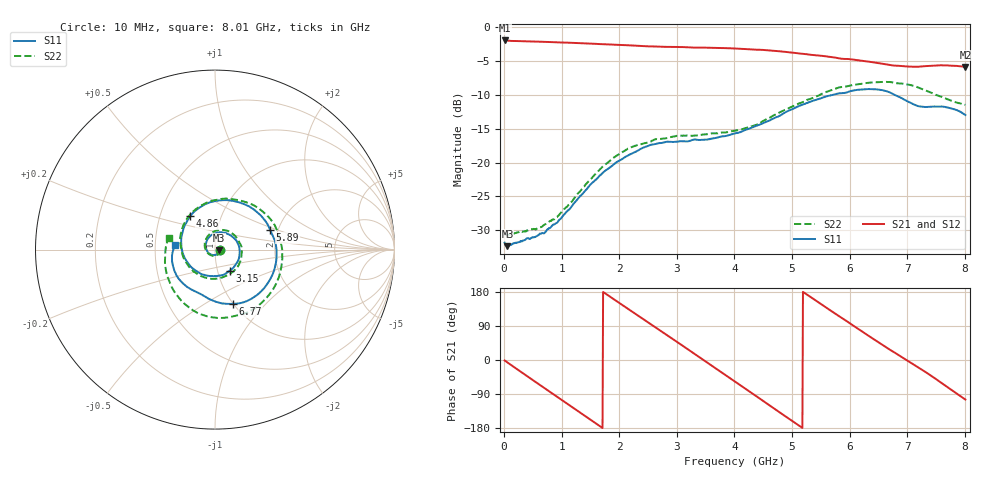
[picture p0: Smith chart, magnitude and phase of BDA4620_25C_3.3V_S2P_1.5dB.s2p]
!Agilent Technologies,E5071B,MY42404982,A.09.10
!Date: Wed May 06 08:56:16 2026
!Data & Calibration Information:
!Freq	S11:SOLT2(ON)	S21:SOLT2(ON)	S12:SOLT2(ON)	S22:SOLT2(ON)
# Hz S RI R 50
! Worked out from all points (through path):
!   801 points, 10 MHz to 8.01 GHz, reference 50 ohm
!   highest |S21| = -1.95 dB at 10 MHz (marker M1); lowest = -5.9 dB at 8.01 GHz (marker M2)
!   group delay of S21, straight-line fit = 286 ps
!   lowest |S11| = -32.3 dB at 60 MHz (marker M3), VSWR 1.05, Z = 52.4 - j0.333 ohm
!   |S11| at or under -10 dB: start of sweep to 5.701 GHz; 6.783 GHz to end of sweep
!   |S22| runs from -30.7 to -8.1 dB; largest |S21 - S12| = 0.0032
!   S11 on the Smith chart (normalised r, x): 10 MHz: 1.05, -0.00; 3.15 GHz: 1.14, -0.28; 4.86 GHz: 0.71, +0.28; 5.89 GHz: 1.81, +0.45; 6.77 GHz: 1.00, -0.67; 8.01 GHz: 0.63, +0.03
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1e7  0.0255 -0.00177  0.7986 -0.017  0.7997 -0.0173  0.0304 -0.002
6e7  0.0239 -0.00318  0.7901 -0.0918  0.7916 -0.0929  0.0289 -0.00346
3.7e8  0.0197 -0.0183  0.609 -0.4991  0.6095 -0.5006  0.0229 -0.0211
7.3e8  -0.00547 -0.0306  0.1729 -0.7596  0.1727 -0.7604  -0.0054 -0.0348
1.03e9  -0.037 -0.017  -0.2455 -0.7308  -0.2462 -0.7319  -0.0401 -0.0197
1.35e9  -0.0517 0.0264  -0.6005 -0.4688  -0.6009 -0.4692  -0.0575 0.0272
1.64e9  -0.0299 0.0723  -0.7452 -0.103  -0.7458 -0.1035  -0.0369 0.0786
1.93e9  0.023 0.0962  -0.688 0.2796  -0.6888 0.2801  0.0197 0.1088
2.32e9  0.1026 0.0669  -0.3374 0.6474  -0.3384 0.6482  0.1091 0.0796
2.68e9  0.1382 -0.0152  0.1146 0.7104  0.1154 0.7111  0.1491 -0.00112
3.15e9  0.0811 -0.1186  0.6002 0.3833  0.6017 0.3825  0.1056 -0.118
3.57e9  -0.0221 -0.1471  0.6924 -0.1315  0.6929 -0.1332  -0.0064 -0.1631
4.01e9  -0.1332 -0.096  0.3816 -0.5824  0.3813 -0.5838  -0.1353 -0.1067
4.42e9  -0.1878 0.0258  -0.1144 -0.6726  -0.1159 -0.6726  -0.1919 0.0273
4.86e9  -0.1384 0.1862  -0.547 -0.3685  -0.5475 -0.3685  -0.1261 0.2082
5.35e9  0.0745 0.2753  -0.5985 0.1789  -0.599 0.1794  0.1076 0.279
5.89e9  0.3071 0.1104  -0.1852 0.5539  -0.1845 0.5549  0.3502 0.0933
6.25e9  0.3338 -0.0994  0.1756 0.5344  0.177 0.5352  0.364 -0.1244
6.68e9  0.1522 -0.2956  0.4614 0.2554  0.4632 0.2551  0.1964 -0.3421
6.77e9  0.0995 -0.3022  0.4872 0.1836  0.4895 0.1834  0.1399 -0.3633
7.35e9  -0.121 -0.2277  0.424 -0.2966  0.4244 -0.2981  -0.1965 -0.2743
8.01e9  -0.2235 0.0234  -0.1263 -0.494  -0.1271 -0.4957  -0.2585 0.066
